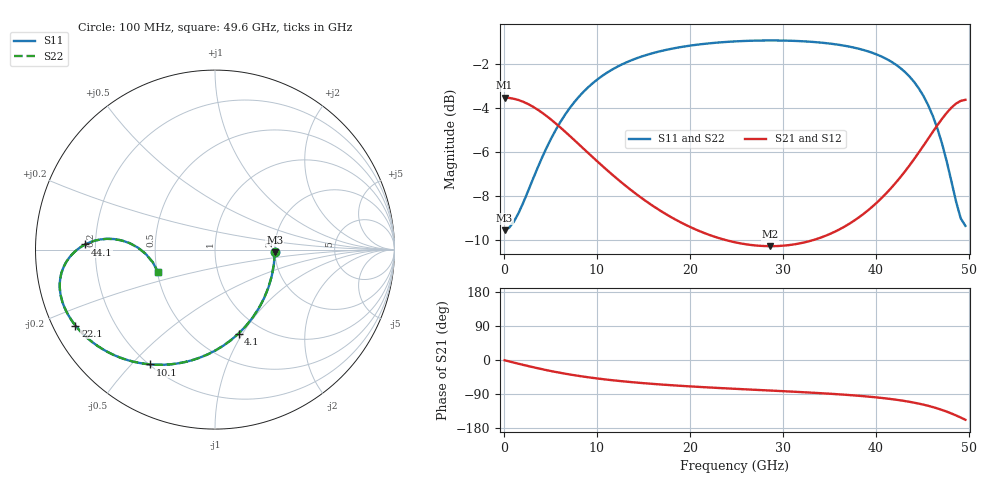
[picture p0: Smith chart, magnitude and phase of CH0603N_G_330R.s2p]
# GHz S RI R 330
! S-Parameters data
! Freq  reS11  imS11  reS21  imS21  reS12  imS12  reS22  imS22
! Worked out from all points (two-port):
!   100 points, 100 MHz to 49.6 GHz, reference 330 ohm
!   highest |S21| = -3.52 dB at 100 MHz (marker M1); lowest = -10.3 dB at 28.6 GHz (marker M2)
!   |S21| within 3 dB of the highest: start of sweep to 10.33 GHz; 43.73 GHz to end of sweep
!   lowest |S11| = -9.5 dB at 100 MHz (marker M3), VSWR 2.00, Z = 659 - j20 ohm
!   |S11| at or under -10 dB: nowhere
!   |S22| runs from -9.5 to -0.9 dB; largest |S21 - S12| = 0
!   S11 on the Smith chart (normalised r, x): 100 MHz: 2.00, -0.06; 4.1 GHz: 0.78, -0.96; 10.1 GHz: 0.20, -0.57; 22.1 GHz: 0.06, -0.25; 44.1 GHz: 0.16, +0.02; 49.6 GHz: 0.50, -0.14
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0.1  0.3332 -0.0135  0.6666 -0.00723  0.6666 -0.00723  0.3332 -0.0135
1.1  0.3164 -0.1466  0.6579 -0.0785  0.6579 -0.0785  0.3164 -0.1466
2.1  0.2736 -0.2707  0.6359 -0.1451  0.6359 -0.1451  0.2736 -0.2707
4.1  0.1311 -0.468  0.5628 -0.252  0.5628 -0.252  0.1311 -0.468
6.1  -0.0446 -0.5855  0.4732 -0.3179  0.4732 -0.3179  -0.0446 -0.5855
7.1  -0.1317 -0.6175  0.4289 -0.3374  0.4289 -0.3374  -0.1317 -0.6175
8.6  -0.2532 -0.6397  0.3674 -0.3537  0.3674 -0.3537  -0.2532 -0.6397
10.1  -0.3596 -0.6398  0.3136 -0.3592  0.3136 -0.3592  -0.3596 -0.6398
13.1  -0.5263 -0.6025  0.2294 -0.3524  0.2294 -0.3524  -0.5263 -0.6025
16.6  -0.6575 -0.5343  0.1624 -0.3345  0.1624 -0.3345  -0.6575 -0.5343
22.1  -0.7777 -0.423  0.0977 -0.3102  0.0977 -0.3102  -0.7777 -0.423
25.1  -0.8164 -0.3663  0.0737 -0.3034  0.0737 -0.3034  -0.8164 -0.3663
28.6  -0.846 -0.3031  0.0503 -0.3026  0.0503 -0.3026  -0.846 -0.3031
33.1  -0.8641 -0.2219  0.0206 -0.3153  0.0206 -0.3153  -0.8641 -0.2219
38.1  -0.8525 -0.1211  -0.027 -0.3548  -0.027 -0.3548  -0.8525 -0.1211
41.6  -0.8045 -0.0357  -0.0935 -0.4044  -0.0935 -0.4044  -0.8045 -0.0357
44.1  -0.7226 0.029  -0.1861 -0.4465  -0.1861 -0.4465  -0.7226 0.029
45.6  -0.6385 0.0566  -0.2759 -0.4615  -0.2759 -0.4615  -0.6385 0.0566
47.1  -0.5208 0.0514  -0.3987 -0.4445  -0.3987 -0.4445  -0.5208 0.0514
48.6  -0.3864 -0.0236  -0.5378 -0.3583  -0.5378 -0.3583  -0.3864 -0.0236
49.1  -0.3477 -0.0692  -0.5779 -0.3091  -0.5779 -0.3091  -0.3477 -0.0692
49.6  -0.3176 -0.1244  -0.6096 -0.2504  -0.6096 -0.2504  -0.3176 -0.1244
